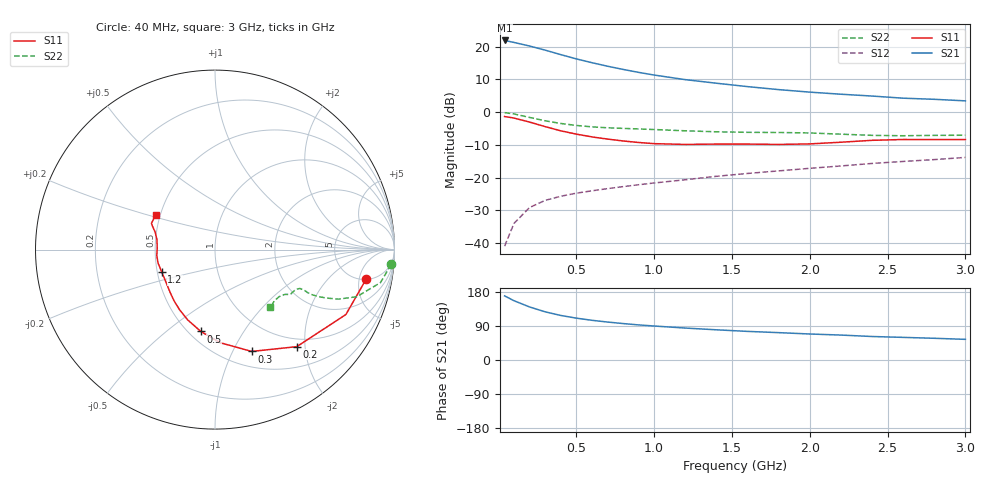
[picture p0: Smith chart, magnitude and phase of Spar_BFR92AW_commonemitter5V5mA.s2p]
! Filename:  BFR92AWB.S2P  Version:  4.0
! NXP part #: BFR92AW  Date: Jun 1994
! Bias condition: Vce=5V, Ic=5mA
#  MHz  S  MA  R  50
! Freq  S11  S21  S12  S22  !GUM [dB]
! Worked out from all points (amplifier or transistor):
!   21 points, 40 MHz to 3 GHz, reference 50 ohm
!   highest |S21| = 21.9 dB at 40 MHz (marker M1)
!   |S21| within 3 dB of that: start of sweep to 303.7 MHz
!   unconditionally stable (mu >= 1): 927 MHz to end of sweep
!   at 300 MHz: K = 0.50, MSG = 22.9 dB, |S12| = -26.9 dB
!   at 1 GHz: K = 1.04, MAG = 15.3 dB, |S12| = -21.6 dB
!   at 3 GHz: K = 1.13, MAG = 6.5 dB, |S12| = -13.8 dB
!   lowest NFmin = 1.60 dB at 500 MHz
!   S11 on the Smith chart (normalised r, x): 40 MHz: 5.15, -6.39; 200 MHz: 0.85, -1.84; 300 MHz: 0.67, -1.19; 500 MHz: 0.57, -0.67; 1.2 GHz: 0.53, -0.15; 3 GHz: 0.47, +0.22
40  0.859 -10.9  12.46 169.2  0.009 83.6  0.985 -4.8
100  0.814 -26.4  11.63 156.5  0.02 74.8  0.94 -11.3
200  0.707 -49.9  10.25 140.0  0.035 64.4  0.832 -18.4
300  0.603 -70.2  8.874 127.2  0.045 58.9  0.74 -21.9
400  0.52 -86.7  7.583 117.6  0.052 56.9  0.673 -23.6
500  0.463 -99.8  6.525 110.5  0.058 56.2  0.628 -24.5
600  0.42 -111.3  5.709 104.8  0.063 57.1  0.598 -24.9
700  0.389 -120.5  5.044 100.2  0.068 58.1  0.578 -24.9
800  0.364 -129.1  4.507 96.2  0.073 59.6  0.566 -24.9
900  0.345 -136.6  4.061 92.6  0.078 60.7  0.555 -24.6
1000  0.331 -143.9  3.695 89.7  0.083 62.0  0.544 -24.5
1200  0.322 -157.0  3.144 84.3  0.093 64.3  0.52 -24.6
1400  0.326 -166.9  2.771 79.7  0.105 66.4  0.502 -26.2
1600  0.326 -174.2  2.46 75.5  0.116 67.9  0.493 -28.7
1800  0.322 178.7  2.213 72.2  0.127 69.9  0.49 -30.2
2000  0.328 170.3  2.026 68.6  0.139 71.4  0.482 -31.2
2200  0.348 163.6  1.882 65.8  0.151 72.3  0.462 -32.7
2400  0.372 159.4  1.765 62.0  0.165 73.1  0.443 -36.3
2600  0.383 157.6  1.637 59.7  0.177 73.7  0.437 -41.0
2800  0.382 154.5  1.574 57.3  0.189 74.8  0.443 -44.3
3000  0.382 149.4  1.49 54.5  0.204 75.3  0.445 -46.3
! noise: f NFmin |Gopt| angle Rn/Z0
500  1.6  0.415  16.9  0.303
1000  2.1  0.286  52.1  0.36
2000  3  0.184  171.9  0.24
